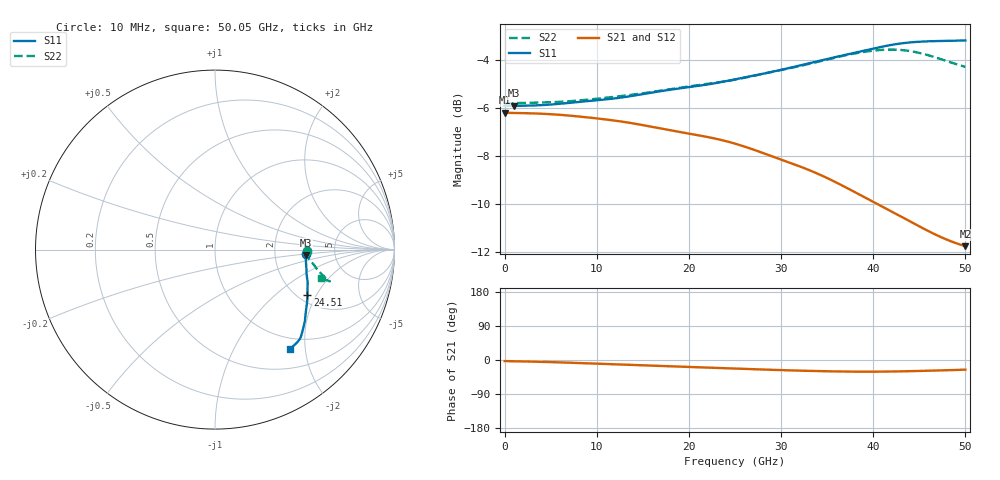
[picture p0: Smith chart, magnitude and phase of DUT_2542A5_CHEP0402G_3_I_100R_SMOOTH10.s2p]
! Touchstone file from project
! Exported from ElectronicsDesktop 2025.1.3
# GHz S MA R 50.000000
! Terminal data exported
! Port[1] = Port1
! Port[2] = Port2
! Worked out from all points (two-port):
!   144 points, 10 MHz to 50.05 GHz, reference 50 ohm
!   highest |S21| = -6.20 dB at 10 MHz (marker M1); lowest = -11.8 dB at 50.05 GHz (marker M2)
!   |S21| within 3 dB of the highest: start of sweep to 36.51 GHz
!   lowest |S11| = -5.9 dB at 1.06 GHz (marker M3), VSWR 3.05, Z = 151 - j12.6 ohm
!   |S11| at or under -10 dB: nowhere
!   |S22| runs from -5.8 to -3.6 dB; largest |S21 - S12| = 0.0037
!   S11 on the Smith chart (normalised r, x): 10 MHz: 3.04, -0.21; 24.51 GHz: 2.25, -1.68; 50.05 GHz: 0.80, -1.71
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0.01  0.5066 -2.9  0.4897 -2.9  0.4892 -2.7  0.5125 -1.1
! Gamma 0 0 0 0
! Port Impedance 50 0 50 0
1.05985  0.5065 -3.5  0.4894 -3.3  0.4888 -3.1  0.513 -1.4
4.2094  0.5084 -5.9  0.4874 -5.0  0.4865 -4.8  0.5147 -2.7
8.4088  0.5167 -10.0  0.4804 -8.2  0.4794 -8.1  0.5202 -4.6
12.6082  0.5268 -14.5  0.4699 -12.0  0.4691 -11.8  0.5307 -6.2
16.8076  0.5429 -18.4  0.4547 -15.6  0.4543 -15.3  0.5442 -7.5
19.95715  0.5536 -21.3  0.4434 -18.3  0.4433 -18.0  0.5556 -8.6
22.4068  0.5626 -23.9  0.4346 -20.4  0.4346 -20.1  0.5638 -9.5
24.5065  0.5723 -26.0  0.4251 -22.2  0.4252 -21.9  0.5719 -10.3
25.2064  0.5759 -26.7  0.4214 -22.8  0.4215 -22.4  0.5752 -10.6
27.65605  0.5886 -29.2  0.4064 -24.8  0.4065 -24.4  0.5883 -11.5
29.75575  0.6002 -31.8  0.393 -26.5  0.3931 -26.1  0.6001 -12.3
31.85545  0.6134 -34.4  0.3799 -28.0  0.38 -27.6  0.6119 -13.1
33.6052  0.625 -36.3  0.3684 -29.0  0.3683 -28.7  0.6228 -13.8
36.05485  0.6407 -38.6  0.3503 -30.2  0.3499 -29.8  0.6394 -14.5
38.5045  0.6563 -41.4  0.3311 -30.8  0.3304 -30.4  0.6538 -15.1
40.25425  0.668 -43.3  0.3178 -30.8  0.317 -30.3  0.6608 -15.3
42.004  0.6785 -44.9  0.3051 -30.4  0.3042 -29.8  0.6635 -15.4
43.4038  0.6848 -46.1  0.2952 -29.8  0.2942 -29.2  0.6613 -15.4
45.15355  0.6893 -47.7  0.2831 -28.9  0.2821 -28.2  0.6523 -15.4
47.95315  0.6919 -50.9  0.2667 -27.1  0.2657 -26.3  0.6286 -15.3
50.05285  0.6933 -53.1  0.2581 -25.5  0.2571 -24.7  0.6105 -15.2
